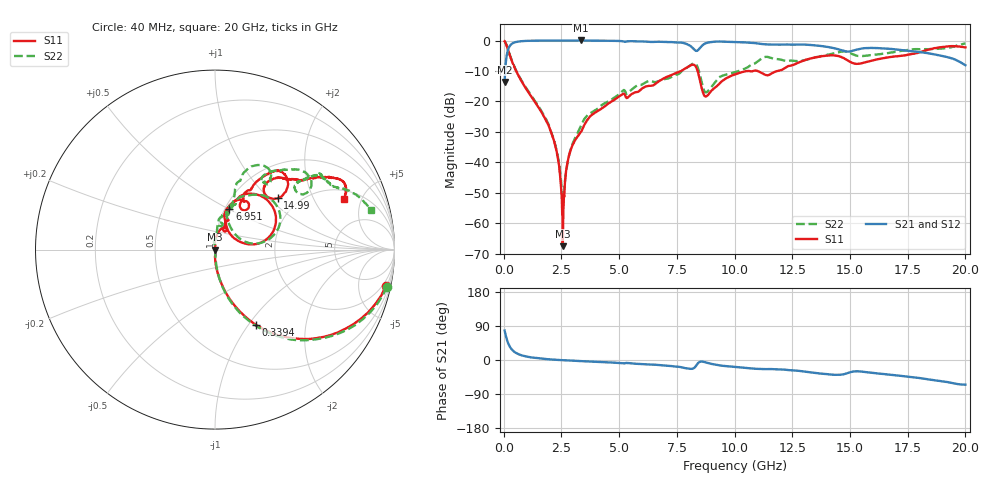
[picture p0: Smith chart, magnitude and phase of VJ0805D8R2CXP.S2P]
! VJ0805D8R2CXP
! DATE 10/29/2021  11:58
! CAPACITORS MOUNTED IN SERIES ON 25 MIL THICK MICROSTRIP SUBSTRATE
# GHz  S  MA  R  50.00
!  FREQ  S11M  S11A  S21M  S21A  S12M  S12A  S22M  S22A
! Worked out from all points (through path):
!   1601 points, 40 MHz to 20 GHz, reference 50 ohm
!   highest |S21| = 0.03 dB at 3.346 GHz (marker M1); lowest = -13.6 dB at 40 MHz (marker M2)
!   group delay of S21, straight-line fit = 9.4 ps
!   lowest |S11| = -67.5 dB at 2.56 GHz (marker M3), VSWR 1.00, Z = 50 - j0.00678 ohm
!   |S11| at or under -10 dB: 539.1 MHz to 7.691 GHz (7.152 GHz wide, 174 % of centre); 8.402 GHz to 10.58 GHz (2.176 GHz wide, 22.9 % of centre); 11 GHz to 11.85 GHz (852.4 MHz wide, 7.46 % of centre)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
!   |S22| runs from -54.0 to -0.2 dB; largest |S21 - S12| = 0.0065
!   S11 on the Smith chart (normalised r, x): 40 MHz: 1.21, -9.36; 339.4 MHz: 1.00, -1.09; 6.951 GHz: 1.05, +0.51; 14.99 GHz: 1.58, +1.13; 20 GHz: 2.55, +3.54
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0.04  0.9734 -12.0  0.208 77.7  0.2081 77.3  0.9829 -12.2
0.1897  0.7013 -45.2  0.7095 44.6  0.7092 44.8  0.7091 -45.4
0.3394  0.4782 -61.4  0.8768 28.6  0.8769 28.6  0.4842 -61.6
0.776025  0.2132 -78.0  0.9768 12.3  0.9771 12.3  0.2194 -78.1
2.036  0.03248 -85.6  0.997 1.5  0.9978 1.4  0.03278 -86.2
2.322925  0.01303 -86.9  0.9976 0.3  0.9975 0.3  0.01405 -80.1
2.55995  0.0004206 -9.3  0.998 -0.5  0.998 -0.5  0.002 -5.0
2.846875  0.0137 84.3  0.999 -1.3  0.9992 -1.4  0.01373 85.2
3.345875  0.03163 91.0  1.004 -2.8  1.004 -2.9  0.03924 97.2
3.370825  0.03258 92.1  1.004 -2.9  1.004 -3.0  0.04125 97.9
5.142275  0.1315 68.1  0.9759 -8.8  0.9762 -8.9  0.1482 81.8
6.70165  0.2119 71.0  0.957 -13.2  0.9566 -13.3  0.2147 70.7
6.95115  0.2414 70.6  0.9496 -14.6  0.9496 -14.7  0.2321 69.0
8.236075  0.4 36.5  0.7239 -21.6  0.7246 -21.7  0.4218 38.5
8.510525  0.2133 7.8  0.7651 -4.5  0.7655 -4.7  0.2654 8.5
8.7725  0.1209 44.4  0.9094 -6.9  0.9098 -7.0  0.1411 40.9
10.02  0.2777 69.3  0.9467 -18.2  0.9471 -18.4  0.3023 69.8
11.32987  0.2736 53.0  0.8658 -24.0  0.8664 -24.1  0.5394 60.4
13.35083  0.515 54.8  0.8429 -33.1  0.8429 -33.5  0.5121 56.1
14.98505  0.4521 39.3  0.661 -32.8  0.6609 -33.0  0.6291 32.5
16.68165  0.5308 48.9  0.7319 -38.6  0.7327 -38.8  0.6236 38.4
20  0.7704 21.4  0.3933 -65.0  0.3929 -65.5  0.8946 14.3
